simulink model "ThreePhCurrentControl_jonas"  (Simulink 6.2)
settings: Solver=ode45  StartTime=0  StopTime=0.05  FixedStep=0.000001  RelTol=1e-3
undefined symbols (not defined in the file or in its folder): di, DiscIntNeverNeededParam, Element, L, R, Sinus, Ts, Udc, Upp, Warning
libraries: simulink x4

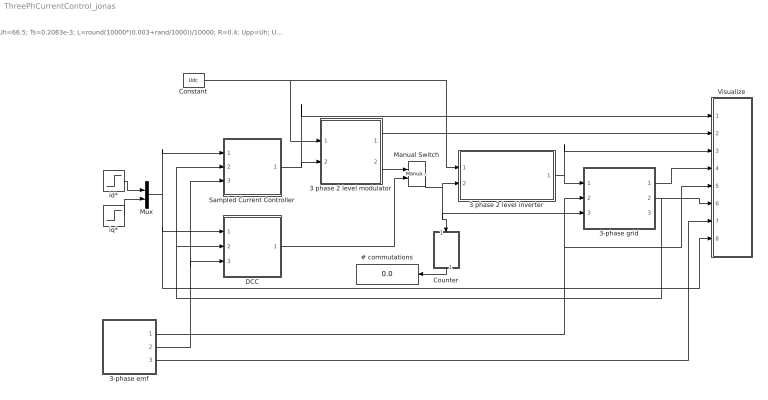
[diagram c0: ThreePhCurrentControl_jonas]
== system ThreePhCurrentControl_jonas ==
  note: Uh=66.5; Ts=0.2083e-3; L=round(10000*(0.003+rand/1000))/10000; R=0.4; Upp=Uh; Udc=250; Cdc=0.0011; di=3; Tf=1/(2*pi*30);
  # commutations : Display
  3 phase 2 level inverter : Subsystem
  3 phase 2 level modulator : Subsystem  mask{type=Sinus, Random=Fixed frequency, Ts=Ts}
      mask prompts: type "Sinus, Symmetrized or Minimum switch modulation"; Random "Fixed or random modulation?"; Ts "Sampling interval"
      mask help: Carrier Wave modulator that uses either fixed frequency modulation or random modulation. The fixed frequency modulation uses 1/(2Ts) as modulation frequency. The random modulation selects the modulatio frequency by random every sampling instant. The selection uses either 1/Ts, 1/(2Ts) or 1/(3Ts) as carrier wave frequency.
  3-phase emf : Subsystem  mask{Upp=Upp, freq=50, Tc=0.1e-3}
      mask prompts: Upp "U_phase_to_phase [RMS]"; freq "Frequency"; Tc "Sampling time"
  3-phase grid : Subsystem  mask{L=L, R=R}
      mask prompts: L "Inductance [H]"; R "Resistance [ohm]"
  Constant : Constant  Value=Udc
  Counter : Subsystem  Orientation=down
  DCC : Subsystem
  Manual Switch : simulink/Signal Routing/Manual Switch  sw=1  action=0
  Mux : Mux  Inputs=2
  Sampled Current Controller : Subsystem  mask{R=R, L=L, Kp=(L/Ts+R/2), Ti=L/R+Ts/2, Ts=Ts, Umax=Udc, Umin=-Udc, SlowFast=Fast computer}
      mask prompts: R "Load resistance"; L "Load inductance"; Kp "Controller gain"; Ti "Integral Time Constant"; Ts "Sampling time [s]"; Umax "Max output signal"; Umin "Min output signal"; SlowFast "Controller type"
  Visualize : Subsystem
  id* : Step  Time=0.0105  After=10  SampleTime=0
  iq* : Step  Time=0.0055  After=10  SampleTime=0
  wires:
  3 phase 2 level inverter/1(va,b,c) -> 3-phase grid/1(va,b,c), Visualize/3(v)
  Sampled Current Controller/1(u*) -> 3 phase 2 level modulator/2(uabc*), Visualize/1(u*)
  Constant/1 -> 3 phase 2 level inverter/1(Udc), 3 phase 2 level modulator/1(Udc)
  Counter/1(#) -> # commutations/1
  3 phase 2 level modulator/2(sa,b,c) -> Manual Switch/1
  Manual Switch/1 -> 3 phase 2 level inverter/2(sa,b,c), Counter/1(sa,b,c), 3-phase grid/3(s)
  DCC/1(sa,b,c) -> Manual Switch/2
  3 phase 2 level modulator/1(mod) -> Visualize/2(mod)
  3-phase emf/1(e_line) -> 3-phase grid/2(e_line), Visualize/5(e)
  3-phase grid/1(u_ab) -> Visualize/4("u ")
  3-phase grid/2(i_ab) -> Visualize/6(i), DCC/2(Act_ab), Sampled Current Controller/2(Act_ab)
  3-phase emf/3(Theta_line) -> Visualize/7(theta)
  3-phase emf/2(Psi_line) -> DCC/3(psi), Sampled Current Controller/3(psi)
  id*/1 -> Mux/1
  iq*/1 -> Mux/2
  Mux/1 -> Sampled Current Controller/1(Ref_dq), DCC/1(Ref_dq), Visualize/8(i*dq)

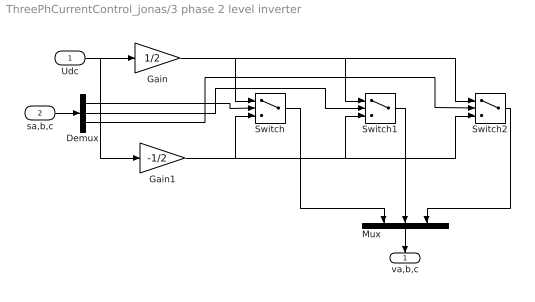
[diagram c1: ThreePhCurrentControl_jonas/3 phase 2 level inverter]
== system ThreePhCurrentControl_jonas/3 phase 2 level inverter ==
  Udc : Inport  Port=1  LatchInput=off
  sa,b,c : Inport  Port=2  LatchInput=off
  Demux : Demux  Outputs=3
  Gain : Gain  Gain=1/2
  Gain1 : Gain  Gain=-1/2
  Mux : Mux  Orientation=down  Inputs=3
  Switch : Switch
  Switch1 : Switch
  Switch2 : Switch
  va,b,c : Outport  Orientation=down  InitialOutput=0
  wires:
  Gain/1 -> Switch/1, Switch1/1, Switch2/1
  Gain1/1 -> Switch/3, Switch1/3, Switch2/3
  Udc/1 -> Gain1/1, Gain/1
  sa,b,c/1 -> Demux/1
  Demux/1 -> Switch/2
  Demux/2 -> Switch1/2
  Demux/3 -> Switch2/2
  Switch/1 -> Mux/1
  Switch1/1 -> Mux/2
  Switch2/1 -> Mux/3
  Mux/1 -> va,b,c/1

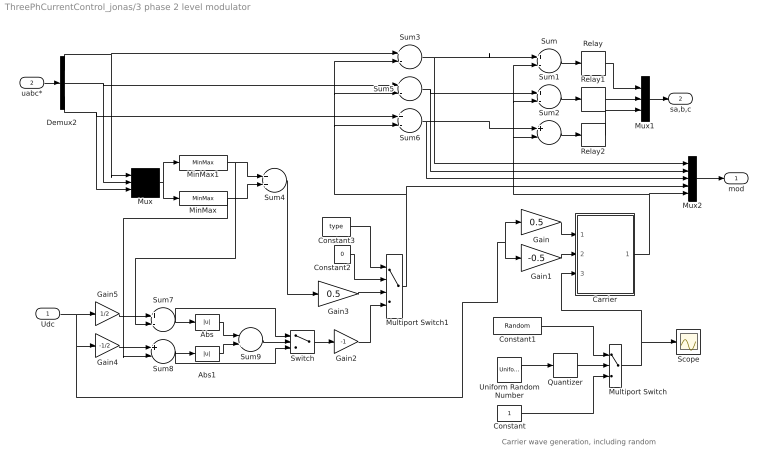
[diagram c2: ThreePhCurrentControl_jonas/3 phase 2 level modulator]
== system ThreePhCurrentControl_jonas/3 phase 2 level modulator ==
  note: Carrier wave generation, including random
  Udc : Inport  Port=1  LatchInput=off
  uabc* : Inport  Port=2  LatchInput=off
  Abs : Abs
  Abs1 : Abs
  Carrier : Subsystem
  Constant : Constant
  Constant1 : Constant  Value=Random
  Constant2 : Constant  Value=0
  Constant3 : Constant  Value=type
  Demux2 : Demux  Outputs=3
  Gain : Gain  Gain=0.5
  Gain1 : Gain  Gain=-0.5
  Gain2 : Gain  Gain=-1
  Gain3 : Gain  Gain=0.5
  Gain4 : Gain  Gain=-1/2
  Gain5 : Gain  Gain=1/2
  MinMax : MinMax
  MinMax1 : MinMax  Function=max
  Multiport Switch : MultiPortSwitch  Inputs=2
  Multiport Switch1 : MultiPortSwitch  Inputs=3
  Mux : Mux  Inputs=3
  Mux1 : Mux  Inputs=3
  Mux2 : Mux  Inputs=5
  Quantizer : Quantizer  QuantizationInterval=1
  Relay : Relay  OffOutputValue=-1
  Relay1 : Relay  OffOutputValue=-1
  Relay2 : Relay  OffOutputValue=-1
  Scope : Scope
  Sum{,1..3,5..8} (8 alike) : Sum  Inputs=+-
  Sum4 : Sum
  Sum9 : Sum  Inputs=-+
  Switch : Switch
  Uniform Random Number : UniformRandomNumber  Minimum=1  Maximum=3  Seed=0.9874  SampleTime=Ts
  mod : Outport  InitialOutput=0
  sa,b,c : Outport  Port=2  InitialOutput=0
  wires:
  Carrier/1(um) -> Sum2/2, Sum1/2, Sum/2, Mux2/5
  Gain1/1 -> Carrier/2(Umin)
  Gain/1 -> Carrier/1(Umax)
  Sum/1 -> Relay/1
  Relay1/1 -> Mux1/2
  Sum1/1 -> Relay1/1
  Relay2/1 -> Mux1/3
  Sum2/1 -> Relay2/1
  Sum3/1 -> Mux2/1, Sum/1
  Sum5/1 -> Mux2/2, Sum1/1
  Sum6/1 -> Mux2/3, Sum2/1
  Demux2/1 -> Sum3/1, Mux/1
  Demux2/2 -> Sum5/1, Mux/2
  Demux2/3 -> Sum6/1, Mux/3
  Mux/1 -> MinMax1/1, MinMax/1
  MinMax1/1 -> Sum4/1, Sum7/2
  MinMax/1 -> Sum4/2, Sum8/2
  Udc/1 -> Gain5/1, Gain4/1, Gain1/1, Gain/1
  Gain4/1 -> Sum8/1
  Sum7/1 -> Abs/1, Switch/1
  Sum8/1 -> Abs1/1, Switch/3
  Abs/1 -> Sum9/1
  Abs1/1 -> Sum9/2
  Sum9/1 -> Switch/2
  Sum4/1 -> Gain3/1
  Switch/1 -> Gain2/1
  Constant3/1 -> Multiport Switch1/1
  Constant2/1 -> Multiport Switch1/2
  Gain3/1 -> Multiport Switch1/3
  Gain2/1 -> Multiport Switch1/4
  Multiport Switch1/1 -> Sum5/2, Sum3/2, Sum6/2, Mux2/4
  Gain5/1 -> Sum7/1
  uabc*/1 -> Demux2/1
  Relay/1 -> Mux1/1
  Mux1/1 -> sa,b,c/1
  Mux2/1 -> mod/1
  Quantizer/1 -> Multiport Switch/2
  Uniform Random Number/1 -> Quantizer/1
  Constant/1 -> Multiport Switch/3
  Multiport Switch/1 -> Scope/1, Carrier/3(x)
  Constant1/1 -> Multiport Switch/1

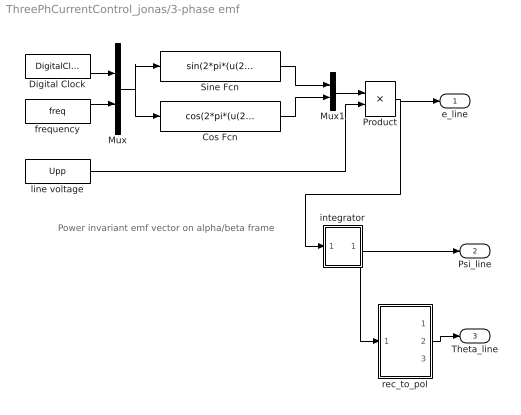
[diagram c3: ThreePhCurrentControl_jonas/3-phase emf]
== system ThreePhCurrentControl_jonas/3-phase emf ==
  note: Power invariant emf vector on alpha/beta frame
  Cos Fcn : Fcn  Expr=cos(2*pi*(u(2))*u(1))
  Digital Clock : DigitalClock  SampleTime=Tc
  Mux : Mux  Inputs=2
  Mux1 : Mux  Inputs=2
  Product : Product
  Sine Fcn : Fcn  Expr=sin(2*pi*(u(2))*u(1)-pi)
  frequency : Constant  Value=freq
  integrator : Subsystem
  line voltage : Constant  Value=Upp
  rec_to_pol : Subsystem
  e_line : Outport  InitialOutput=0
  Psi_line : Outport  Port=2  InitialOutput=0
  Theta_line : Outport  Port=3  InitialOutput=0
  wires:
  Product/1 -> e_line/1, integrator/1(In1)
  Mux1/1 -> Product/1
  Cos Fcn/1 -> Mux1/2
  Sine Fcn/1 -> Mux1/1
  Mux/1 -> Cos Fcn/1, Sine Fcn/1
  Digital Clock/1 -> Mux/1
  frequency/1 -> Mux/2
  line voltage/1 -> Product/2
  integrator/1(Out1) -> Psi_line/1, rec_to_pol/1(rect)
  rec_to_pol/2(angle) -> Theta_line/1

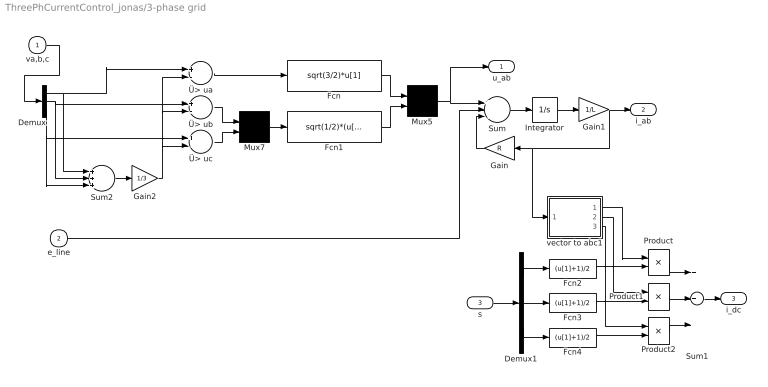
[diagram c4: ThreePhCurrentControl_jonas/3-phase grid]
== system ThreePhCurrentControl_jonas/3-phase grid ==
  va,b,c : Inport  Port=1  LatchInput=off
  e_line : Inport  Port=2  LatchInput=off
  s : Inport  Port=3  LatchInput=off
  Demux : Demux  Outputs=3
  Demux1 : Demux  Outputs=3
  Fcn : Fcn  Expr=sqrt(3/2)*u[1]
  Fcn1 : Fcn  Expr=sqrt(1/2)*(u[1]-u[2])
  Fcn2 : Fcn  Expr=(u[1]+1)/2
  Fcn3 : Fcn  Expr=(u[1]+1)/2
  Fcn4 : Fcn  Expr=(u[1]+1)/2
  Gain : Gain  Orientation=left  Gain=R
  Gain1 : Gain  Gain=1/L
  Gain2 : Gain  Gain=1/3
  Integrator : Integrator
  Mux5 : Mux  Inputs=2
  Mux7 : Mux  Inputs=2
  Product : Product
  Product1 : Product
  Product2 : Product
  Sum : Sum  Inputs=+--
  Sum1 : Sum  Inputs=+++
  Sum2 : Sum  Inputs=+++
  vector to abc1 : Subsystem
  Ü> ua : Sum  Inputs=+-
  Ü> ub : Sum  Inputs=+-
  Ü> uc : Sum  Inputs=+-
  u_ab : Outport  InitialOutput=0
  i_ab : Outport  Port=2  InitialOutput=0
  i_dc : Outport  Port=3
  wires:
  Gain1/1 -> i_ab/1, Gain/1, vector to abc1/1(vect)
  Integrator/1 -> Gain1/1
  Gain/1 -> Sum/3
  Sum/1 -> Integrator/1
  Fcn1/1 -> Mux5/2
  Fcn/1 -> Mux5/1
  Mux5/1 -> Sum/1, u_ab/1
  Mux7/1 -> Fcn1/1
  Ü> uc/1 -> Mux7/2
  Ü> ub/1 -> Mux7/1
  Ü> ua/1 -> Fcn/1
  Gain2/1 -> Ü> uc/2, Ü> ub/2, Ü> ua/2
  Demux/2 -> Ü> ub/1, Sum2/2
  Sum2/1 -> Gain2/1
  Demux/3 -> Ü> uc/1, Sum2/3
  Demux/1 -> Ü> ua/1, Sum2/1
  va,b,c/1 -> Demux/1
  Demux1/2 -> Fcn3/1
  Demux1/1 -> Fcn2/1
  Demux1/3 -> Fcn4/1
  s/1 -> Demux1/1
  Sum1/1 -> i_dc/1
  Product2/1 -> Sum1/3
  Product1/1 -> Sum1/2
  Product/1 -> Sum1/1
  vector to abc1/1(a) -> Product/1
  vector to abc1/2(b) -> Product1/1
  vector to abc1/3(c) -> Product2/1
  Fcn4/1 -> Product2/2
  Fcn3/1 -> Product1/2
  Fcn2/1 -> Product/2
  e_line/1 -> Sum/2

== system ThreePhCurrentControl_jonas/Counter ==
  sa,b,c : Inport  Port=1  LatchInput=off
  Demux : Demux  Outputs=3
  Subsystem : Subsystem  TreatAsAtomicUnit=on
  Subsystem1 : Subsystem  TreatAsAtomicUnit=on
  Subsystem2 : Subsystem  TreatAsAtomicUnit=on
  Sum : Sum  Inputs=+++
  # : Outport
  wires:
  Sum/1 -> #/1
  Subsystem/1(Out1) -> Sum/2
  Subsystem2/1(Out1) -> Sum/1
  Subsystem1/1(Out1) -> Sum/3
  sa,b,c/1 -> Demux/1
  Demux/2 -> Subsystem/Trigger
  Demux/3 -> Subsystem1/Trigger
  Demux/1 -> Subsystem2/Trigger

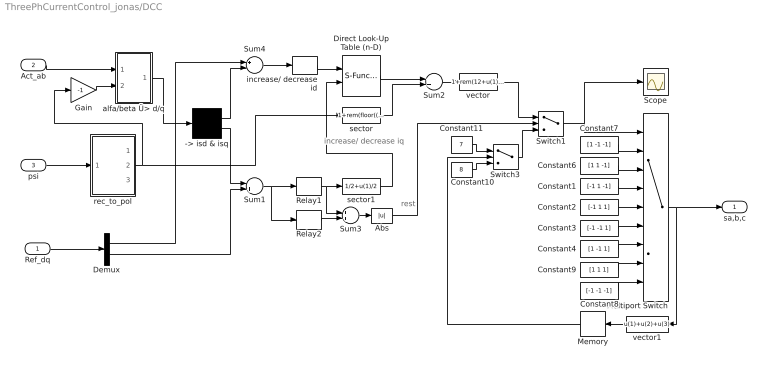
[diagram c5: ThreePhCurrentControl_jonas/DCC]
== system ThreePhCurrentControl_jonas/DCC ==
  note: increase/ decrease iq
  note: rest
  Ref_dq : Inport  Port=1  LatchInput=off
  Act_ab : Inport  Port=2  LatchInput=off
  psi : Inport  Port=3  LatchInput=off
  -> isd & isq : Demux  Outputs=2
  Abs : Abs
  Constant1 : Constant  Value=[-1 1 -1]
  Constant10 : Constant  Value=8
  Constant11 : Constant  Value=7
  Constant2 : Constant  Value=[-1 1 1]
  Constant3 : Constant  Value=[-1 -1 1]
  Constant4 : Constant  Value=[1 -1 1]
  Constant6 : Constant  Value=[1 1 -1]
  Constant7 : Constant  Value=[1 -1 -1]
  Constant8 : Constant  Value=[-1 -1 -1]
  Constant9 : Constant  Value=[1 1 1]
  Demux : Demux  Outputs=2
  Direct Look-Up Table (n-D) : S-Function  FunctionName=sfun_nddirectlook  Parameters=numInputs,mxTable,clipFlag,tabIsInput,numTDims  mask(LookupNDDirect){maskTabDims=2, explicitNumDims=1, outDims=Element, tabIsInput=off, mxTable=[4 2;5 1], clipFlag=Warning}
      mask prompts: maskTabDims "Number of table dimensions:"; explicitNumDims "Explicit number of table dimensions:"; outDims "Inputs select this object from table:"; tabIsInput "Make table an input"; mxTable "Table data:"; clipFlag "Action for out of range input:"
      mask help: Table member selection. Inputs are zero-based indices into the table, e.g., an input of 3 returns the fourth element in that dimension. Block can also be used to select a column or 2-D matrix out of the table.
      mask init:
      | if tabIsInput == 1
      |   tWhat = ' T';
      |   yT = 1/(3+maskTabDims-outDims);
      | else
      |   tWhat = ' ';
      |   yT = 0;
      | end
      | if maskTabDims >= 5
      |   numTDims = explicitNumDims;
      | else
      |   numTDims = maskTabDims;
      | end
      | numInputs =  numTDims - (outDims-1);
      | if strcmp(get_param(bdroot(gcb),'BlockDiagramType'),'library')
      |   dimsChar = 'n';
      | else
      |   dimsChar = sprintf('%d',numTDims);
      | end
      | [x,y] = nddirectico('plotdata', numTDims, tabIsInput, outDims);
      | xp = x((end-3):end); yp = y((end-3):end);
      | x = x(1:(end-4)); y = y(1:(end-4));
  Gain : Gain  Gain=-1
  Memory : Memory  Orientation=left
  Multiport Switch : MultiPortSwitch  Inputs=8
  Relay1 : Relay  OnSwitchValue=di/2  OffSwitchValue=-di/2  OffOutputValue=-1
  Relay2 : Relay  OnSwitchValue=1.3*di/2  OffSwitchValue=-1.3*di/2  OffOutputValue=-1
  Scope : Scope
  Sum1 : Sum  Inputs=-+
  Sum2 : Sum
  Sum3 : Sum
  Sum4 : Sum  Inputs=+-
  Switch1 : Switch  Threshold=1
  Switch3 : Switch  Threshold=1
  alfa/beta Ü> d/q : Subsystem
  increase/ decrease id : Relay  OnSwitchValue=di/2  OffSwitchValue=-di/2
  rec_to_pol : Subsystem
  sector : Fcn  Expr=1+rem(floor((2*pi+u(1)+pi/6)/(pi/3+eps)),6)
  sector1 : Fcn  Expr=1/2+u(1)/2
  vector : Fcn  Expr=1+rem(12+u(1)-1,6)
  vector1 : Fcn  Orientation=left  Expr=u(1)+u(2)+u(3)
  sa,b,c : Outport
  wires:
  Gain/1 -> alfa/beta Ü> d/q/2(angle)
  Act_ab/1 -> alfa/beta Ü> d/q/1(vect)
  alfa/beta Ü> d/q/1(Out) -> -> isd & isq/1
  psi/1 -> rec_to_pol/1(rect)
  -> isd & isq/1 -> Sum4/2
  rec_to_pol/2(angle) -> Gain/1, sector/1
  Multiport Switch/1 -> vector1/1, sa,b,c/1
  Switch1/1 -> Multiport Switch/1, Scope/1
  vector/1 -> Switch1/1
  Sum4/1 -> increase/ decrease id/1
  Sum2/1 -> vector/1
  vector1/1 -> Memory/1
  -> isd & isq/2 -> Sum1/1
  Constant10/1 -> Switch3/3
  Constant11/1 -> Switch3/1
  Memory/1 -> Switch3/2
  Switch3/1 -> Switch1/3
  Relay1/1 -> Sum3/1, sector1/1
  Relay2/1 -> Sum3/2
  Sum3/1 -> Abs/1
  Sum1/1 -> Relay1/1, Relay2/1
  Abs/1 -> Switch1/2
  increase/ decrease id/1 -> Direct Look-Up Table (n-D)/1
  sector1/1 -> Direct Look-Up Table (n-D)/2
  sector/1 -> Sum2/2
  Direct Look-Up Table (n-D)/1 -> Sum2/1
  Constant6/1 -> Multiport Switch/3
  Constant7/1 -> Multiport Switch/2
  Constant8/1 -> Multiport Switch/9
  Constant9/1 -> Multiport Switch/8
  Constant1/1 -> Multiport Switch/4
  Constant2/1 -> Multiport Switch/5
  Constant3/1 -> Multiport Switch/6
  Constant4/1 -> Multiport Switch/7
  Ref_dq/1 -> Demux/1
  Demux/1 -> Sum4/1
  Demux/2 -> Sum1/2

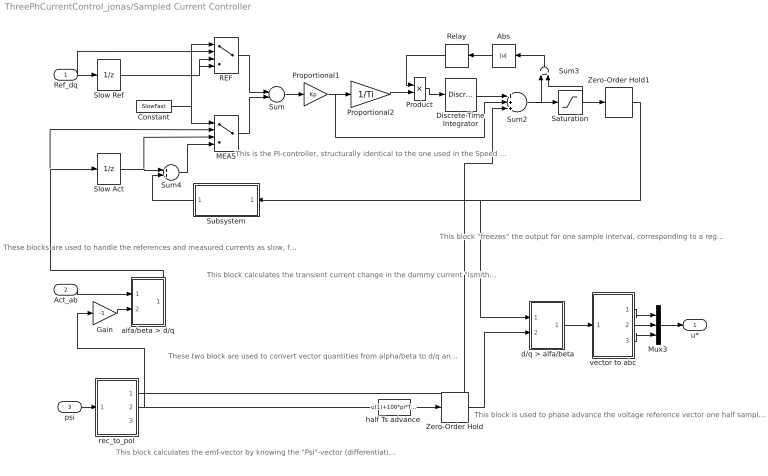
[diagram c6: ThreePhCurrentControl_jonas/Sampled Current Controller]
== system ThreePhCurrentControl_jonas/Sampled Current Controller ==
  note: These blocks are used to handle the references and measured currents as slow, fast or fast computer with Smith predictor.
  note: This block calculates the transient current change in the dummy current "ismith" The smith predictor calculates the current change that would have been measured if the computer was "fast", i.e. without the delay that a slow computer has. The calculated current change equals the real current change, but informing the controller one sampling interval earlier, thus allowing a high (deadbeat) gain.
  note: This is the PI-controller, structurally identical to the one used in the Speed Controller
  note: This block "freezes" the output for one sample interval, corresponding to a register in a microcontroller where the reference voltages are written once every sampling inteval.
  note: These two block are used to convert vector quantities from alpha/beta to d/q and back again. Note that they are identical, but use the angle with opposite sign.
  note: This block calculates the emf-vector by knowing the "Psi"-vector (differentiation) and calculates the emf- components in the d/q-plane (ideally there is only "eq" whilse "ed"=0). It alse calculates the angle of the "Psi"- vector, used to orient the d/q-plane.
  note: This block is used to phase advance the voltage reference vector one half sample period. It is done to compensate for the fact that the "reality" is turning during the same sample period as the voltage references are being held constant. In the beginning of the sample period, the voltage reference will be 1/2 sample period ahead of reality, and in the end of the sample period it will be 1/2 period behind. In average, it will be in the correct position relative to reality.
  Ref_dq : Inport  Port=1  LatchInput=off
  Act_ab : Inport  Port=2  LatchInput=off
  psi : Inport  Port=3  LatchInput=off
  " d/q > alfa/beta" : Subsystem
  Abs : Abs  Orientation=left
  Constant : Constant  Value=SlowFast
  Discrete-Time Integrator : DiscreteIntegrator  SampleTime=Ts  LimitOutput=on  UpperSaturationLimit=Umax  LowerSaturationLimit=Umin  ICPrevOutput=DiscIntNeverNeededParam  ICPrevScaledInput=DiscIntNeverNeededParam
  Gain : Gain  Gain=-1
  MEAS : MultiPortSwitch  Inputs=3
  Mux3 : Mux  Inputs=3
  Product : Product
  Proportional1 : Gain  Gain=Kp
  Proportional2 : Gain  Gain=1/Ti
  REF : MultiPortSwitch  Inputs=3
  Relay : Relay  Orientation=left  OnOutputValue=0  OffOutputValue=1
  Saturation : Saturate  UpperLimit=Umax  LowerLimit=Umin
  Slow Act : UnitDelay  SampleTime=Ts
  Slow Ref : UnitDelay  SampleTime=Ts
  Subsystem : Subsystem  Orientation=left
  Sum : Sum  Inputs=+-
  Sum2 : Sum  Inputs=+++
  Sum3 : Sum  Orientation=up  Inputs=+-
  Sum4 : Sum
  Zero-Order Hold : ZeroOrderHold  SampleTime=Ts
  Zero-Order Hold1 : ZeroOrderHold  SampleTime=Ts
  alfa/beta > d/q : Subsystem
  "half Ts advance " : Fcn  Expr=u(1)+100*pi*Ts/2
  rec_to_pol : Subsystem
  vector to abc : Subsystem
  u* : Outport
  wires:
  Discrete-Time Integrator/1 -> Sum2/1
  Proportional1/1 -> Proportional2/1, Sum2/2
  Sum/1 -> Proportional1/1
  Sum2/1 -> Saturation/1, Sum3/1
  Saturation/1 -> Zero-Order Hold1/1, Sum3/2
  Proportional2/1 -> Product/2
  Product/1 -> Discrete-Time Integrator/1
  Relay/1 -> Product/1
  Ref_dq/1 -> REF/2, Slow Ref/1
  Zero-Order Hold1/1 -> Subsystem/1(u), " d/q > alfa/beta"/1(vect)
  Slow Act/1 -> Sum4/1, MEAS/3
  Subsystem/1(di_smith) -> Sum4/2
  Constant/1 -> MEAS/1, REF/1
  Slow Ref/1 -> REF/3, REF/4
  REF/1 -> Sum/1
  Sum4/1 -> MEAS/4
  MEAS/1 -> Sum/2
  Sum3/1 -> Abs/1
  Abs/1 -> Relay/1
  Gain/1 -> alfa/beta > d/q/2(angle)
  Act_ab/1 -> alfa/beta > d/q/1(vect)
  psi/1 -> rec_to_pol/1(rect)
  rec_to_pol/2(angle) -> Gain/1, "half Ts advance "/1
  "half Ts advance "/1 -> Zero-Order Hold/1
  Zero-Order Hold/1 -> " d/q > alfa/beta"/2(angle)
  " d/q > alfa/beta"/1(Out) -> vector to abc/1(vect)
  vector to abc/1(a) -> Mux3/1
  vector to abc/2(b) -> Mux3/2
  vector to abc/3(c) -> Mux3/3
  alfa/beta > d/q/1(Out) -> Slow Act/1, MEAS/2
  Mux3/1 -> u*/1
  rec_to_pol/1(e) -> Sum2/3

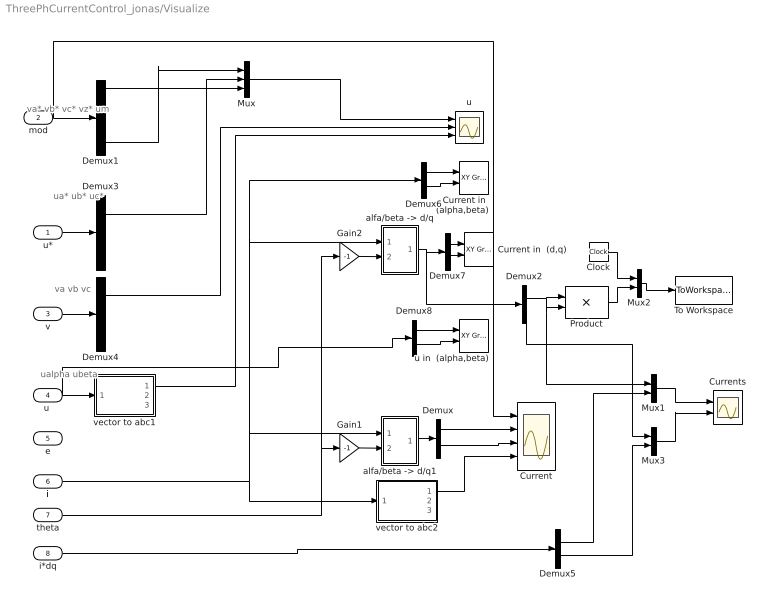
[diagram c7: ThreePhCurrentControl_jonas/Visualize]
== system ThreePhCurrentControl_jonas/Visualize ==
  note: va* vb* vc* vz* um
  note: ua* ub* uc*
  note: ualpha ubeta
  note: va vb vc
  u* : Inport  Port=1  LatchInput=off
  mod : Inport  Port=2  LatchInput=off
  v : Inport  Port=3  LatchInput=off
  "u " : Inport  Port=4  LatchInput=off
  e : Inport  Port=5  LatchInput=off
  i : Inport  Port=6  LatchInput=off
  theta : Inport  Port=7  LatchInput=off
  i*dq : Inport  Port=8  LatchInput=off
  Clock : Clock
  Current : Scope  NumInputPorts=4
  Current in  (alpha,beta) : simulink/Sinks/XY Graph  xmin=-20  xmax=20  ymin=-20  ymax=20  st=-1
  Current in  (d,q) : simulink/Sinks/XY Graph  xmin=-20  xmax=20  ymin=-20  ymax=20  st=-1
  Currents : Scope  NumInputPorts=2
  Demux{,2,5..8} (6 alike) : Demux  Outputs=2
  Demux1 : Demux  Outputs=5
  Demux3 : Demux  Outputs=3
  Demux4 : Demux  Outputs=3
  Gain1 : Gain  Gain=-1
  Gain2 : Gain  Gain=-1
  Mux : Mux  Inputs=3
  Mux1 : Mux  Inputs=2
  Mux2 : Mux  Inputs=2
  Mux3 : Mux  Inputs=2
  Product : Product
  To Workspace : ToWorkspace  VariableName=f1  SampleTime=-1  SaveFormat=Array
  "alfa/beta -> d/q" : Subsystem
  "alfa/beta -> d/q1" : Subsystem
  u : Scope  NumInputPorts=3
  u in  (alpha,beta) : simulink/Sinks/XY Graph  xmin=-300  xmax=300  ymin=-300  ymax=300  st=-1
  vector to abc1 : Subsystem
  vector to abc2 : Subsystem
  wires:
  Gain2/1 -> "alfa/beta -> d/q"/2(angle)
  Gain1/1 -> "alfa/beta -> d/q1"/2(angle)
  "alfa/beta -> d/q1"/1(Out) -> Demux/1
  Demux/1 -> Current/2
  Demux/2 -> Current/3
  vector to abc2/1(a) -> Current/4
  mod/1 -> Demux1/1, Current/1
  "alfa/beta -> d/q"/1(Out) -> Demux2/1, Demux7/1
  Demux1/5 -> Mux/1
  Demux1/1 -> Mux/3
  Mux/1 -> u/1
  u*/1 -> Demux3/1
  "u "/1 -> vector to abc1/1(vect), Demux8/1
  Demux3/1 -> Mux/2
  v/1 -> Demux4/1
  Demux4/1 -> u/2
  vector to abc1/1(a) -> u/3
  i/1 -> "alfa/beta -> d/q"/1(vect), Demux6/1, "alfa/beta -> d/q1"/1(vect), vector to abc2/1(vect)
  e/1 -> ?
  theta/1 -> Gain1/1, Gain2/1
  Clock/1 -> Mux2/1
  Product/1 -> Mux2/2
  Mux2/1 -> To Workspace/1
  Demux2/1 -> Product/1, Product/2, Mux1/1
  i*dq/1 -> Demux5/1
  Demux5/1 -> Mux1/2
  Demux2/2 -> Mux3/1
  Demux5/2 -> Mux3/2
  Mux3/1 -> Currents/2
  Mux1/1 -> Currents/1
  Demux6/1 -> Current in  (alpha,beta)/1
  Demux6/2 -> Current in  (alpha,beta)/2
  Demux7/1 -> Current in  (d,q)/1
  Demux7/2 -> Current in  (d,q)/2
  Demux8/1 -> u in  (alpha,beta)/1
  Demux8/2 -> u in  (alpha,beta)/2

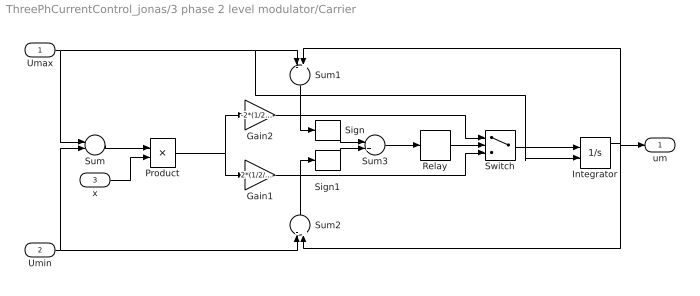
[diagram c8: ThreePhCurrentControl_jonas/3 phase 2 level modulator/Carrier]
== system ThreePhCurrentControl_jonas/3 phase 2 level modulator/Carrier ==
  Umax : Inport  Port=1  LatchInput=off
  Umin : Inport  Port=2  LatchInput=off
  x : Inport  Port=3  LatchInput=off
  Gain1 : Gain  Gain=2*(1/2/Ts)
  Gain2 : Gain  Gain=-2*(1/2/Ts)
  Integrator : Integrator  InitialConditionSource=external
  Product : Product
  Relay : Relay  OnSwitchValue=1  OffSwitchValue=-1  OffOutputValue=-1
  Sign : Signum
  Sign1 : Signum
  Sum : Sum  Inputs=+-
  Sum1 : Sum  Orientation=down  Inputs=-+
  Sum2 : Sum  Orientation=up  Inputs=-+
  Sum3 : Sum
  Switch : Switch
  um : Outport
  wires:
  Switch/1 -> Integrator/1
  Umax/1 -> Sum/1, Sum1/1, Integrator/2
  Umin/1 -> Sum/2, Sum2/1
  Gain2/1 -> Switch/1
  Gain1/1 -> Switch/3
  Integrator/1 -> Sum1/2, um/1, Sum2/2
  Sum1/1 -> Sign/1
  Sum2/1 -> Sign1/1
  Sign/1 -> Sum3/1
  Sign1/1 -> Sum3/2
  Sum3/1 -> Relay/1
  Relay/1 -> Switch/2
  Sum/1 -> Product/1
  Product/1 -> Gain2/1, Gain1/1
  x/1 -> Product/2

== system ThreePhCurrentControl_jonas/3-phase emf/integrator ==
  note: Power invariant emf vector on alpha/beta frame
  In1 : Inport  Port=1  LatchInput=off
  Demux : Demux  Outputs=2
  Integrator1 : Integrator  InitialCondition=Upp/(2*pi*freq)
  Integrator2 : Integrator
  Mux : Mux  Inputs=2
  Out1 : Outport
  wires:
  In1/1 -> Demux/1
  Mux/1 -> Out1/1
  Integrator2/1 -> Mux/2
  Integrator1/1 -> Mux/1
  Demux/2 -> Integrator2/1
  Demux/1 -> Integrator1/1

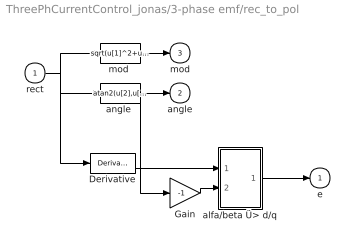
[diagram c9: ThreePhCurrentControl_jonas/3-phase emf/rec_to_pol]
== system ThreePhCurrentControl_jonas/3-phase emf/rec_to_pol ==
  rect : Inport  Port=1  LatchInput=off
  Derivative : Derivative
  Gain : Gain  Gain=-1
  alfa/beta Ü> d/q : Subsystem
  "angle " : Fcn  Expr=atan2(u[2],u[1])
  "mod " : Fcn  Expr=sqrt(u[1]^2+u[2]^2)
  e : Outport  InitialOutput=0
  angle : Outport  Port=2  InitialOutput=0
  mod : Outport  Port=3  InitialOutput=0
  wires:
  "angle "/1 -> angle/1, Gain/1
  rect/1 -> "angle "/1, "mod "/1, Derivative/1
  "mod "/1 -> mod/1
  Gain/1 -> alfa/beta Ü> d/q/2(angle)
  Derivative/1 -> alfa/beta Ü> d/q/1(vect)
  alfa/beta Ü> d/q/1(Out) -> e/1

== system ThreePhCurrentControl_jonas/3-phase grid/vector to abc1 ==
  vect : Inport  Port=1  LatchInput=off
  Ü> a : Fcn  Expr=sqrt(2/3)*u[1]
  Ü> b : Fcn  Expr=-sqrt(1/6)*u[1]+sqrt(1/2)*u[2]
  Ü> c : Fcn  Expr=-sqrt(1/6)*u[1]-sqrt(1/2)*u[2]
  a : Outport  InitialOutput=0
  b : Outport  Port=2  InitialOutput=0
  c : Outport  Port=3  InitialOutput=0
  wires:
  vect/1 -> Ü> b/1, Ü> a/1, Ü> c/1
  Ü> b/1 -> b/1
  Ü> c/1 -> c/1
  Ü> a/1 -> a/1

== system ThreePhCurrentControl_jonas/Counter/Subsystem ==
  Trigger : TriggerPort  TriggerType=either
  Constant : Constant
  Memory : Memory  Orientation=left  InheritSampleTime=on
  Sum : Sum
  Out1 : Outport
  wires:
  Sum/1 -> Memory/1, Out1/1
  Memory/1 -> Sum/2
  Constant/1 -> Sum/1

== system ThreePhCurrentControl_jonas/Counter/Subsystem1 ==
  Trigger : TriggerPort  TriggerType=either
  Constant : Constant
  Memory : Memory  Orientation=left  InheritSampleTime=on
  Sum : Sum
  Out1 : Outport
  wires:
  Constant/1 -> Sum/1
  Memory/1 -> Sum/2
  Sum/1 -> Memory/1, Out1/1

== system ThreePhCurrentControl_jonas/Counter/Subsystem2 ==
  Trigger : TriggerPort  TriggerType=either
  Constant : Constant
  Memory : Memory  Orientation=left  InheritSampleTime=on
  Sum : Sum
  Out1 : Outport
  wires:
  Sum/1 -> Memory/1, Out1/1
  Memory/1 -> Sum/2
  Constant/1 -> Sum/1

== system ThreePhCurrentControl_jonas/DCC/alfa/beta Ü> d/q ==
  vect : Inport  Port=1  LatchInput=off
  angle : Inport  Port=2  LatchInput=off
  Fcn : Fcn  Expr=u[1]*cos(u[3])-u[2]*sin(u[3])
  Fcn1 : Fcn  Expr=u[1]*sin(u[3])+u[2]*cos(u[3])
  Mux : Mux  Inputs=2
  Mux1 : Mux  Inputs=2
  Out : Outport  InitialOutput=0
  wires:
  vect/1 -> Mux/1
  angle/1 -> Mux/2
  Mux/1 -> Fcn/1, Fcn1/1
  Fcn/1 -> Mux1/1
  Fcn1/1 -> Mux1/2
  Mux1/1 -> Out/1

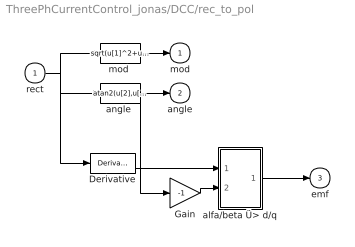
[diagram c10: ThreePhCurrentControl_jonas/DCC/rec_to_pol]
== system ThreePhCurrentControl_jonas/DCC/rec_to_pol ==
  rect : Inport  Port=1  LatchInput=off
  Derivative : Derivative
  Gain : Gain  Gain=-1
  alfa/beta Ü> d/q : Subsystem
  "angle " : Fcn  Expr=atan2(u[2],u[1])
  "mod " : Fcn  Expr=sqrt(u[1]^2+u[2]^2)
  mod : Outport  InitialOutput=0
  angle : Outport  Port=2  InitialOutput=0
  emf : Outport  Port=3  InitialOutput=0
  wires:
  "angle "/1 -> angle/1, Gain/1
  rect/1 -> "angle "/1, "mod "/1, Derivative/1
  "mod "/1 -> mod/1
  Gain/1 -> alfa/beta Ü> d/q/2(angle)
  Derivative/1 -> alfa/beta Ü> d/q/1(vect)
  alfa/beta Ü> d/q/1(Out) -> emf/1

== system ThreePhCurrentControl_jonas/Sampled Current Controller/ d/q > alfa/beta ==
  vect : Inport  Port=1  LatchInput=off
  angle : Inport  Port=2  LatchInput=off
  Fcn : Fcn  Expr=u[1]*cos(u[3])-u[2]*sin(u[3])
  Fcn1 : Fcn  Expr=u[1]*sin(u[3])+u[2]*cos(u[3])
  Mux : Mux  Inputs=2
  Mux1 : Mux  Inputs=2
  Out : Outport  InitialOutput=0
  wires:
  Mux1/1 -> Out/1
  Fcn1/1 -> Mux1/2
  Fcn/1 -> Mux1/1
  Mux/1 -> Fcn1/1, Fcn/1
  angle/1 -> Mux/2
  vect/1 -> Mux/1

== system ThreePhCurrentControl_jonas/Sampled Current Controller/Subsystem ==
  u : Inport  Orientation=left  Port=1  LatchInput=off
  Gammalt mätvärde2 : UnitDelay  Orientation=down  SampleTime=Ts
  Gammalt mätvärde3 : UnitDelay  Orientation=left  SampleTime=Ts
  Matsprediktor1 : Sum  Orientation=left  Inputs=+-
  Proportional3 : Gain  Orientation=left  Gain=Ts/L
  Proportional4 : Gain  Orientation=left  Gain=(1-Ts/(L/R))
  Sum1 : Sum  Orientation=left
  di_smith : Outport  Orientation=left
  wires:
  Proportional3/1 -> Sum1/1
  Proportional4/1 -> Sum1/2
  Sum1/1 -> Gammalt mätvärde2/1, Matsprediktor1/1
  u/1 -> Proportional3/1
  Matsprediktor1/1 -> Gammalt mätvärde3/1
  Gammalt mätvärde3/1 -> di_smith/1
  Gammalt mätvärde2/1 -> Proportional4/1, Matsprediktor1/2

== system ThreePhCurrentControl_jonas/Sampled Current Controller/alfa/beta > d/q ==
  vect : Inport  Port=1  LatchInput=off
  angle : Inport  Port=2  LatchInput=off
  Fcn : Fcn  Expr=u[1]*cos(u[3])-u[2]*sin(u[3])
  Fcn1 : Fcn  Expr=u[1]*sin(u[3])+u[2]*cos(u[3])
  Mux : Mux  Inputs=2
  Mux1 : Mux  Inputs=2
  Out : Outport  InitialOutput=0
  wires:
  vect/1 -> Mux/1
  angle/1 -> Mux/2
  Mux/1 -> Fcn/1, Fcn1/1
  Fcn/1 -> Mux1/1
  Fcn1/1 -> Mux1/2
  Mux1/1 -> Out/1

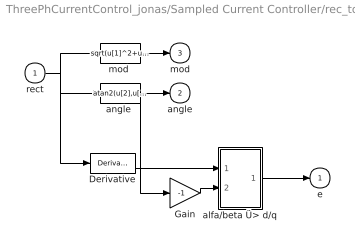
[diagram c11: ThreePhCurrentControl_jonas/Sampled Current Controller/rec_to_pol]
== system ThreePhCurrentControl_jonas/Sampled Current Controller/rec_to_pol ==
  rect : Inport  Port=1  LatchInput=off
  Derivative : Derivative
  Gain : Gain  Gain=-1
  alfa/beta Ü> d/q : Subsystem
  "angle " : Fcn  Expr=atan2(u[2],u[1])
  "mod " : Fcn  Expr=sqrt(u[1]^2+u[2]^2)
  e : Outport  InitialOutput=0
  angle : Outport  Port=2  InitialOutput=0
  mod : Outport  Port=3  InitialOutput=0
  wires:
  "angle "/1 -> angle/1, Gain/1
  rect/1 -> "angle "/1, "mod "/1, Derivative/1
  "mod "/1 -> mod/1
  Gain/1 -> alfa/beta Ü> d/q/2(angle)
  Derivative/1 -> alfa/beta Ü> d/q/1(vect)
  alfa/beta Ü> d/q/1(Out) -> e/1

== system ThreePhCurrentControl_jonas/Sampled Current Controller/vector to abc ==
  vect : Inport  Port=1  LatchInput=off
  Ü> a : Fcn  Expr=sqrt(2/3)*u[1]
  Ü> b : Fcn  Expr=-sqrt(1/6)*u[1]+sqrt(1/2)*u[2]
  Ü> c : Fcn  Expr=-sqrt(1/6)*u[1]-sqrt(1/2)*u[2]
  a : Outport  InitialOutput=0
  b : Outport  Port=2  InitialOutput=0
  c : Outport  Port=3  InitialOutput=0
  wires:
  vect/1 -> Ü> b/1, Ü> a/1, Ü> c/1
  Ü> b/1 -> b/1
  Ü> c/1 -> c/1
  Ü> a/1 -> a/1

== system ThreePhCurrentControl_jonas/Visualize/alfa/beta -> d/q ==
  vect : Inport  Port=1  LatchInput=off
  angle : Inport  Port=2  LatchInput=off
  Fcn : Fcn  Expr=u[1]*cos(u[3])-u[2]*sin(u[3])
  Fcn1 : Fcn  Expr=u[1]*sin(u[3])+u[2]*cos(u[3])
  Mux : Mux  Inputs=2
  Mux1 : Mux  Inputs=2
  Out : Outport  InitialOutput=0
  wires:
  vect/1 -> Mux/1
  angle/1 -> Mux/2
  Mux/1 -> Fcn/1, Fcn1/1
  Fcn/1 -> Mux1/1
  Fcn1/1 -> Mux1/2
  Mux1/1 -> Out/1

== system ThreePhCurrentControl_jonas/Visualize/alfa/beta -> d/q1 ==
  vect : Inport  Port=1  LatchInput=off
  angle : Inport  Port=2  LatchInput=off
  Fcn : Fcn  Expr=u[1]*cos(u[3])-u[2]*sin(u[3])
  Fcn1 : Fcn  Expr=u[1]*sin(u[3])+u[2]*cos(u[3])
  Mux : Mux  Inputs=2
  Mux1 : Mux  Inputs=2
  Out : Outport  InitialOutput=0
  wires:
  Mux1/1 -> Out/1
  Fcn1/1 -> Mux1/2
  Fcn/1 -> Mux1/1
  Mux/1 -> Fcn1/1, Fcn/1
  angle/1 -> Mux/2
  vect/1 -> Mux/1

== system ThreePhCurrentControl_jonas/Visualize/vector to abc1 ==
  vect : Inport  Port=1  LatchInput=off
  Ü> a : Fcn  Expr=sqrt(2/3)*u[1]
  Ü> b : Fcn  Expr=-sqrt(1/6)*u[1]+sqrt(1/2)*u[2]
  Ü> c : Fcn  Expr=-sqrt(1/6)*u[1]-sqrt(1/2)*u[2]
  a : Outport  InitialOutput=0
  b : Outport  Port=2  InitialOutput=0
  c : Outport  Port=3  InitialOutput=0
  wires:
  Ü> a/1 -> a/1
  Ü> c/1 -> c/1
  Ü> b/1 -> b/1
  vect/1 -> Ü> c/1, Ü> a/1, Ü> b/1

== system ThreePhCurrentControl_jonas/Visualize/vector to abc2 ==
  vect : Inport  Port=1  LatchInput=off
  Ü> a : Fcn  Expr=sqrt(2/3)*u[1]
  Ü> b : Fcn  Expr=-sqrt(1/6)*u[1]+sqrt(1/2)*u[2]
  Ü> c : Fcn  Expr=-sqrt(1/6)*u[1]-sqrt(1/2)*u[2]
  a : Outport  InitialOutput=0
  b : Outport  Port=2  InitialOutput=0
  c : Outport  Port=3  InitialOutput=0
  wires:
  vect/1 -> Ü> b/1, Ü> a/1, Ü> c/1
  Ü> b/1 -> b/1
  Ü> c/1 -> c/1
  Ü> a/1 -> a/1

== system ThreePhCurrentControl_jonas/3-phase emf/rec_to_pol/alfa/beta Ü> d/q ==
  vect : Inport  Port=1  LatchInput=off
  angle : Inport  Port=2  LatchInput=off
  Fcn : Fcn  Expr=u[1]*cos(u[3])-u[2]*sin(u[3])
  Fcn1 : Fcn  Expr=u[1]*sin(u[3])+u[2]*cos(u[3])
  Mux : Mux  Inputs=2
  Mux1 : Mux  Inputs=2
  Out : Outport  InitialOutput=0
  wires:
  vect/1 -> Mux/1
  angle/1 -> Mux/2
  Mux/1 -> Fcn/1, Fcn1/1
  Fcn/1 -> Mux1/1
  Fcn1/1 -> Mux1/2
  Mux1/1 -> Out/1

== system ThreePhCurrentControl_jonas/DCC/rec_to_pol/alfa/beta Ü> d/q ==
  vect : Inport  Port=1  LatchInput=off
  angle : Inport  Port=2  LatchInput=off
  Fcn : Fcn  Expr=u[1]*cos(u[3])-u[2]*sin(u[3])
  Fcn1 : Fcn  Expr=u[1]*sin(u[3])+u[2]*cos(u[3])
  Mux : Mux  Inputs=2
  Mux1 : Mux  Inputs=2
  Out : Outport  InitialOutput=0
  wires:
  vect/1 -> Mux/1
  angle/1 -> Mux/2
  Mux/1 -> Fcn/1, Fcn1/1
  Fcn/1 -> Mux1/1
  Fcn1/1 -> Mux1/2
  Mux1/1 -> Out/1

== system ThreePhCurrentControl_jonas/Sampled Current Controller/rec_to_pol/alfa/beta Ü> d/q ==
  vect : Inport  Port=1  LatchInput=off
  angle : Inport  Port=2  LatchInput=off
  Fcn : Fcn  Expr=u[1]*cos(u[3])-u[2]*sin(u[3])
  Fcn1 : Fcn  Expr=u[1]*sin(u[3])+u[2]*cos(u[3])
  Mux : Mux  Inputs=2
  Mux1 : Mux  Inputs=2
  Out : Outport  InitialOutput=0
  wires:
  vect/1 -> Mux/1
  angle/1 -> Mux/2
  Mux/1 -> Fcn/1, Fcn1/1
  Fcn/1 -> Mux1/1
  Fcn1/1 -> Mux1/2
  Mux1/1 -> Out/1
